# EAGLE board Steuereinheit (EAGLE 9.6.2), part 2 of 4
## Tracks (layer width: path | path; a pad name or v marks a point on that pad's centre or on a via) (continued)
GND  (via drill 0.35)  (1 unrouted) (continued)
  Top 0.152: SE_JK2.8 SE_JK2.7 17.7,55.35 17.7,54.63 16.81,53.75 v15.57,53.75 | v15.75,45.57 18.06,45.57 18.95,44.68 18.95,43.97 BR_NO3.8 | SE_JK7.8 18.95,101.22 17.88,101.22 SE_JK7.7 17.7,101.04 17.7,99.8 16.64,98.73 v15.57,98.73 | v17.53,97.49 18.06,97.49 18.95,96.6 18.95,95.88 SE_JK6.9 | v16.28,108.86 18.06,108.86 18.95,107.97 18.95,107.26 SE_JK7.9 | SE_JK12.7 17.88,66.9 18.95,66.9 SE_JK12.8 19.13,66.9 21.62,66.9 23.75,69.04 23.75,70.64 21.62,72.77 19.13,72.77 SE_JK12.9 18.95,72.95 18.95,73.66 18.06,74.55 v15.57,74.55 | v15.57,79.88 18.95,83.26 18.95,84.33 SE_JK5.9 | PL_XR.11 42.6,24.77 43.66,24.77 PL_XR.10 43.84,24.77 43.84,25.3 44.2,25.65 | 44.2,25.65 46.33,27.79 46.33,29.92 M_OR1.7 | PL_XR.7 46.33,18.36 46.33,17.83 45.62,17.12 43.31,17.12 42.6,17.83 42.6,18.36 PL_XR.4 42.6,18.54 42.6,19.25 v43.48,20.14 | v43.48,26.37 44.2,25.65 | v44.2,56.95 45.97,56.95 46.86,56.06 46.86,55.35 BR_AA4.7 | 52.38,108.69 52.55,108.86 SE_BF1.3 52.38,108.69 | 52.38,108.69 50.95,107.26 50.95,105.13 52.2,103.89 52.55,103.89 SE_BF2.3 | 52.55,112.6 52.55,112.06 51.66,111.18 51.66,109.4 52.38,108.69 | 52.55,112.6 52.55,113.84 SE_BF0.3 | SE_AN2.7 48.28,101.22 48.82,101.75 50.06,101.75 50.42,101.4 50.42,100.15 51.66,98.91 52.55,98.91 SE_BF3.3 52.55,98.73 v52.55,97.84 | v52.73,77.39 52.73,78.28 SE_BF7.3 | v52.73,112.6 52.55,112.6 | SE_JK10.12 30.51,95.88 30.51,96.42 31.22,97.13 33.53,97.13 34.24,96.42 34.24,95.88 SE_JK10.9 34.24,95.71 34.24,91.97 | SE_JK9.12 30.51,84.33 30.51,83.62 31.22,82.91 33.53,82.91 34.24,83.62 34.24,84.33 SE_JK9.9 34.24,84.51 34.24,85.22 31.75,87.71
  Top 0.152: SE_JK6.7 17.88,89.66 18.95,89.66 SE_JK6.8 19.13,89.48 21.08,89.48 23.39,87.17 28.91,87.17 29.26,87.53 | 29.26,87.53 29.26,89.48 SE_JK10.4 | 29.26,87.53 29.62,87.17 v30.86,87.17 31.22,87.17 31.75,87.71 | 31.75,87.71 32.99,88.95 32.99,89.48 SE_JK10.7 33.17,89.66 34.24,89.66 | 34.24,89.66 34.24,91.97 | 34.24,89.66 SE_JK10.8 | BR_NO4.8 48.28,66.9 48.28,70.99 49.35,72.06 49.35,77.04 48.28,78.1 SE_JK8.8 48.11,78.28 47.04,78.28 SE_JK8.7 46.86,78.28 46.86,78.99 46.15,79.7 44.55,79.7 | 52.55,88.42 52.2,88.06 | 52.2,88.06 50.77,86.64 50.77,84.86 52.02,83.62 52.55,83.62 SE_BF6.3 | 51.31,91.44 52.55,92.69 52.55,93.57 SE_BF4.3 | 51.31,91.44 51.31,89.66 52.55,88.42 | 52.55,88.42 SE_BF5.3 | 48.28,85.75 48.28,89.48 SE_AN1.7 48.11,89.66 48.11,90.37 46.68,91.8 46.68,92.86 47.22,93.4 48.82,93.4 50.77,91.44 51.31,91.44 | 48.28,85.75 48.28,84.51 SE_JK8.9 | SE_JK9.7 33.17,78.28 34.24,78.28 SE_JK9.8 34.42,78.1 35.66,78.1 | 44.55,79.7 44.02,79.7 43.31,78.99 43.31,78.28 SE_JK8.4 43.13,78.1 43.13,77.57 42.06,76.5 38.68,76.5 37.08,78.1 35.66,78.1 | 44.55,79.7 44.55,84.33 SE_JK8.12 44.55,84.51 44.55,85.04 45.26,85.75 48.28,85.75 | 34.24,91.97 35.31,91.97 35.66,91.62 35.66,78.1 | 52.2,88.06 v52.73,87.53 | X2.M2 9.53,8.59 X2.M3 9.35,8.76 9.35,10.01 7.04,12.32 C9.1 6.86,12.5 5.79,13.56 5.79,17.12 9.17,20.5 10.06,20.5 FT232.7 | 18.95,18.19 19.66,18.19 20.19,18.72 20.19,19.43 19.66,19.96 18.95,19.96 | 18.95,18.19 17.88,18.19 FT232.18 | 18.95,19.96 17.88,19.96 FT232.21 | 18.95,19.96 18.95,22.28 18.77,22.45 17.88,22.45 FT232.25 17.88,22.63 17.88,23.16 FT232.26 17.7,23.34 v15.39,23.34
  Top 0.152: X2.M1 18.41,8.59 X2.M4 | X2.5 15.57,8.76 18.41,8.76 X2.M4 | 18.95,13.74 18.95,9.12 18.59,8.76 X2.M4 | 18.95,13.74 18.95,18.19 | X2.M1 X2.M2 | X2.M2 | X2.M1 | 31.75,18.54 32.46,19.25 32.99,19.25 | 32.99,19.25 33.53,19.25 34.24,18.54 34.24,18.01 SE_N01.8 | SE_JK1.7 17.88,30.1 18.95,30.1 SE_JK1.8 19.13,29.92 21.08,29.92 25.53,25.48 26.06,25.48 26.77,24.77 | 26.77,24.77 26.77,24.05 SE_N01.15 26.77,24.77 | 26.77,24.77 27.48,25.48 29.62,25.48 30.33,24.77 | 30.33,24.77 30.33,24.05 SE_N01.12 30.33,24.77 | 31.04,25.48 32.28,25.48 32.99,24.77 32.99,24.05 SE_N01.10 32.99,23.88 32.99,19.25 | 30.33,24.77 31.04,25.48 | 30.86,27.61 26.77,27.61 22.86,31.52 22.86,34.54 21.44,35.97 19.13,35.97 SE_JK1.9 | 30.86,27.61 33.35,27.61 34.24,28.5 34.24,29.92 SE_AN3.7 | CLKNO.7 46.86,12.14 29.79,12.14 29.26,12.68 MCLKC.2 29.08,12.85 28.19,13.74 18.95,13.74 | v30.86,27.96 30.86,27.61 | v30.86,25.65 31.04,25.48 | 31.75,102.46 32.28,102.46 32.99,101.75 32.99,101.22 SE_JK11.7 33.17,101.22 34.24,101.22 SE_JK11.8 | 31.75,102.46 29.97,102.46 29.26,101.75 29.26,101.22 SE_JK11.4 | SE_JK11.9 34.24,107.09 34.24,106.55 33.53,105.84 31.22,105.84 30.51,106.55 30.51,107.09 SE_JK11.12 30.51,107.26 v30.51,108.86 | v31.75,102.82 31.75,102.46 | SE_JK5.7 17.88,78.28 18.95,78.28 SE_JK5.8 19.13,78.1 20.55,78.1 22.68,75.97 27.66,75.97 28.91,77.22 | 28.91,77.22 29.08,77.39 29.08,78.1 SE_JK9.4 28.91,77.22 | SE_JK3.7 SE_JK3.8 34.42,55.35 34.42,61.39 SE_JK3.9 34.24,61.57 34.24,62.1 32.64,63.7 v30.86,63.7 | SE_JK4.8 34.24,66.9 33.17,66.9 SE_JK4.7 32.99,66.9 v32.99,68.5 | v31.57,42.19 33.17,42.19 34.24,43.26 34.24,43.79 BR_OR1.7
  Top 0.152: v32.99,71.17 33.17,71.17 34.24,72.24 34.24,72.77 SE_JK4.9 | v29.62,76.5 28.91,77.22 | BR_JK4.7 144.3,45.21 145.36,45.21 BR_JK4.8 145.54,45.21 145.54,47.35 | 145.54,47.35 145.54,51.26 BR_JK4.9 | 141.45,42.01 140.39,43.08 140.39,45.03 BR_JK4.4 140.39,45.21 140.39,46.99 141.45,48.06 | 141.45,42.01 141.45,40.06 BR_JK8.12 141.45,39.88 141.45,37.57 139.14,35.26 | 141.45,48.06 141.45,51.26 BR_JK4.12 | 145.54,47.35 142.16,47.35 141.45,48.06 | BR_JK7.12 127.76,40.06 127.76,40.59 128.47,41.3 130.61,41.3 131.32,40.59 131.32,40.06 BR_JK7.9 131.32,39.88 131.32,37.74 129.72,36.14 | 127.23,35.26 128.12,36.14 129.72,36.14 | 127.23,35.26 126.52,34.54 126.52,33.83 BR_JK7.4 | 129.72,36.14 130.07,35.79 130.07,33.83 BR_JK7.7 130.25,33.83 131.32,33.83 BR_JK7.8 131.5,33.83 134.7,33.83 136.12,35.26 139.14,35.26 | BR_JK8.9 145.54,39.88 145.54,33.83 BR_JK8.8 145.36,33.83 144.3,33.83 BR_JK8.7 144.12,33.66 144.12,33.12 143.41,32.41 141.1,32.41 140.39,33.12 140.39,33.66 BR_JK8.4 140.21,33.83 140.21,34.54 139.5,35.26 139.14,35.26 | 144.83,82.02 144.83,82.55 145.54,83.26 145.54,88.77 144.83,89.48 PC_AN10.7 | 144.83,82.02 144.83,78.28 PC_AN11.7 | v142.88,99.44 143.76,99.44 144.65,100.33 144.65,101.04 PC_AN5.7 | 144.83,82.02 142.7,82.02 v141.99,82.73 | 138.43,67.44 137.72,68.15 136.65,68.15 135.41,66.9 130.96,66.9 PC_AN8.7 | 138.43,67.44 PC_NO1.2 138.43,66.9 | 140.92,67.44 140.92,66.9 PC_NO1.4 140.92,67.44 | 140.92,67.44 140.21,68.15 139.14,68.15 138.43,67.44 | v142.52,56.95 142.52,57.12 143.23,57.84 144.12,57.84 145.9,56.06 145.9,55.35 PC_NO2.8 | v142.52,63.35 143.23,63.35 145.9,66.02 145.9,66.73 PC_NO1.8
  Top 0.152: 140.92,67.44 141.99,68.5 v142.52,68.5 | v141.99,42.01 141.45,42.01 | v145.36,22.45 144.83,22.99 144.83,23.7 RE_BF3.3 | v132.21,22.63 132.21,23.7 WR_BF3.3 | 145.36,13.74 144.83,13.74 RE_BF1.3 145.36,13.74 | 145.36,13.74 145.9,14.28 145.9,17.65 144.83,18.72 RE_BF2.3 | 132.21,3.25 132.21,8.41 WR_BF0.3 | 132.21,3.25 133.99,1.47 139.68,1.47 141.1,2.9 141.1,5.03 144.65,8.59 RE_BF0.3 144.83,8.59 145.19,8.59 145.9,9.3 145.9,10.72 145.36,11.25 145.36,12.32 | 125.81,2.54 125.81,6.45 132.03,12.68 132.03,13.56 WR_BF1.3 | 125.81,2.54 126.52,1.83 130.78,1.83 132.21,3.25 | 132.03,16.94 132.03,18.72 WR_BF2.3 | 132.03,16.94 123.32,8.23 123.32,2.54 | 123.32,2.54 124.03,1.83 125.09,1.83 125.81,2.54 | 123.32,2.54 122.61,1.83 119.05,1.83 118.16,2.72 118.16,7.52 126.87,16.23 126.87,18.36 BR_AN2.7 | 145.36,12.32 145.36,13.74 | 132.03,16.94 v132.21,16.94 | 145.36,12.32 v145.54,12.32 | 129.18,102.82 129.72,102.82 130.78,101.75 130.78,101.22 PC_AN9.7 | 129.18,102.82 122.96,102.82 121.36,101.22 115.67,101.22 PC_JK5.8 115.49,101.22 115.49,101.75 114.43,102.82 v113,102.82 | v128.12,91.26 129.9,91.26 130.78,90.37 130.78,89.66 PC_AN6.7 | v129.18,103.18 129.18,102.82 | BR_JK3.4 126.34,45.21 126.34,48.95 127.58,50.19 127.58,51.26 BR_JK3.12 127.76,51.44 127.76,52.15 128.3,52.68 | BR_JK3.7 130.25,45.21 131.32,45.21 BR_JK3.8 131.5,45.21 131.5,51.26 BR_JK3.9 131.32,51.44 130.96,51.79 130.96,52.68 | 130.96,52.68 130.96,55.35 PC_AN1.7 | 130.96,52.68 128.3,52.68 | v127.94,76.33 129.54,76.33 130.78,77.57 130.78,78.1 PC_AN7.7 | v127.94,53.04 128.3,52.68 | 127.23,35.26 127.05,35.26 v126.87,35.43 | 98.25,51.08 98.6,51.44 100.91,51.44
  Top 0.152: 98.25,51.08 97.89,50.72 97.89,50.19 BR_JK2.12 | 100.91,51.44 101.45,50.9 101.45,50.19 BR_JK2.9 101.45,50.01 101.45,46.99 99.67,45.21 | 100.91,51.44 101.45,51.97 101.45,55.35 BR_NO1.8 | BR_JK1.12 85.09,48.59 85.98,47.7 87.76,47.7 88.82,48.77 | 88.82,48.77 88.82,50.01 BR_JK1.9 | 99.67,45.21 100.2,44.68 100.2,43.97 BR_JK2.7 100.38,43.97 101.45,43.97 BR_JK2.8 | 99.67,45.21 99.49,45.39 97.36,45.39 96.65,44.68 96.65,43.97 BR_JK2.4 96.47,43.79 96.47,43.26 95.4,42.19 92.02,42.19 91.67,42.55 91.67,45.92 88.82,48.77 | v99.85,91.26 100.56,91.26 101.45,90.37 101.45,89.66 PC_JK2.8 | v99.31,103 100.38,103 101.45,101.93 101.45,101.22 PC_JK1.8 | BR_NO1.2 93.98,56.06 96.11,58.19 | 96.11,58.19 97,59.08 101.09,59.08 102.34,60.33 102.34,64.77 PC_AN3.7 | 97.89,37.03 97.89,38.63 BR_JK6.12 | 97.89,37.03 98.6,36.32 99.85,36.32 101.45,37.92 101.45,38.63 BR_JK6.9 | v97,20.14 97.71,20.85 99.49,20.85 100.2,20.14 100.2,18.54 BR_AN4.7 | v97.54,37.03 97.89,37.03 | 96.11,58.19 97.36,56.95 v97.54,56.95 | 98.25,51.08 97.71,51.61 v97.71,51.79 | BR_OR7.11 111.23,38.63 111.23,39.34 v112.12,40.23 113.72,41.83 115.85,41.83 116.74,42.72 116.74,52.15 115.67,53.21 115.67,55.35 PC_AN4.7 | 112.47,22.99 112.47,21.57 114.78,19.25 114.78,18.54 BR_AN7.7 | 112.47,22.99 112.47,24.59 BR_AN7.10 | BR_OR6.7 115.49,43.79 115.49,43.26 114.78,42.55 112.47,42.55 111.76,43.26 BR_OR6.4 111.76,45.21 v112.12,45.57 | v112.12,22.99 112.47,22.99 | v114.96,91.26 115.49,90.73 115.49,89.66 PC_JK6.8 | PC_JK3.8 101.62,78.1 103.94,78.1 106.07,75.97 118.16,75.97 118.87,76.68 118.87,77.39 118.16,78.1 115.67,78.1 PC_JK7.8 115.49,78.28 115.49,78.99 114.61,79.88 v112.12,79.88
  Top 0.152: v112.12,68.5 114.43,68.5 115.49,67.44 115.49,66.9 PC_JK4.8 | BR_JK5.12 85.09,37.92 85.62,37.39 | 85.62,37.39 85.8,37.21 88.11,37.21 88.82,37.92 88.82,38.63 BR_JK5.9 89,38.63 89,43.79 | 96.65,33.3 96.65,32.59 BR_JK6.4 | 96.65,33.3 97.18,33.83 99.67,33.83 100.2,33.3 100.2,32.59 BR_JK6.7 100.38,32.59 101.45,32.59 BR_JK6.8 101.62,32.41 103.05,30.99 111.58,30.99 112.65,29.92 114.96,29.92 115.32,30.28 115.32,30.99 114.96,31.34 114.96,32.41 BR_OR7.7 114.78,32.59 114.78,33.3 113.89,34.19 v112.12,34.19 | 89,43.79 90.25,43.79 90.78,43.26 90.78,39.52 92.02,38.28 92.02,36.86 93.45,35.43 94.51,35.43 96.65,33.3 | 89,43.79 BR_JK1.8 | 96.65,33.3 BR_JK6.4 | 84.73,20.85 85.98,20.85 87.58,19.25 87.58,18.54 BR_AN3.7 | 84.73,20.85 80.29,20.85 77.98,18.54 74.95,18.54 BR_OR4.7 | v84.73,20.14 84.73,20.85 | 85.62,37.39 85.62,37.21 v85.45,37.03 | v58.06,68.5 58.78,69.22 59.66,69.22 60.91,67.97 60.91,66.9 BR_OR2.7 | v56.29,16.76 58.6,16.76 59.66,17.83 59.66,18.36 M_NO1.8 | BR_JK5.8 88.82,32.59 87.76,32.59 BR_JK5.7 87.58,32.59 87.58,33.12 86.87,33.83 84.56,33.83 83.84,33.12 83.84,32.59 BR_JK5.4 83.67,32.41 83.67,30.63 | 77.44,31.7 80.11,29.03 83.31,29.03 83.67,29.39 83.67,30.63 | 77.44,31.7 76.73,32.41 76.2,32.41 BR_NO2.8 | 47.04,45.57 47.04,43.97 BR_AA1.7 | 47.04,45.57 47.57,46.1 49.53,46.1 49.89,45.75 59.13,45.75 59.66,46.28 60.38,46.28 60.91,45.75 | 60.91,45.75 60.91,43.97 BR_AA2.7 61.09,43.79 61.09,41.83 62.86,40.06 PLC.2 62.86,34.54 67.31,30.1 v72.11,30.1 75.84,30.1 77.44,31.7 | 60.91,45.75 62.51,47.35 62.51,47.52 62.69,47.7 62.69,51.08 61.09,52.68 61.09,55.35 BR_AA3.7
  Top 0.152: 66.06,111.71 66.06,110.82 SP_BF1.3 | 66.06,111.71 68.02,113.66 68.02,114.38 66.6,115.8 66.06,115.8 SP_BF0.3 | v65.53,81.66 65.89,81.31 65.89,80.42 SP_BF7.3 | v64.82,86.64 65.89,85.57 SP_BF6.3 | 66.06,111.71 65.53,111.71 v65.18,112.06 | 67.67,97.31 66.06,95.71 SP_BF4.3 | 67.67,99.44 67.67,97.31 | 67.67,99.44 66.6,100.51 66.06,100.51 SP_BF3.3 | 67.67,99.44 69.09,100.86 69.09,103 66.42,105.66 66.06,105.66 SP_BF2.3 65.89,105.84 64.82,106.91 v63.58,106.91 | 87.58,87.88 69.98,87.88 67.49,90.37 66.06,90.37 SP_BF5.3 | 87.58,87.88 88.11,88.42 88.11,89.84 86.51,91.44 M48Z08.20 84.56,91.44 81,95 70.51,95 68.2,97.31 67.67,97.31 | 86.87,65.3 87.58,66.02 87.58,66.73 PC_AN2.7 | 86.87,65.3 86.51,64.95 81.36,64.95 81,64.59 78.87,64.59 76.73,66.73 74.95,66.73 BR_AN6.7 | 74.95,45.57 74.95,46.99 78.16,50.19 78.16,51.08 79.76,52.68 82.25,52.68 82.42,52.86 87.05,52.86 87.58,53.39 87.58,55.17 BR_OR5.7 87.76,55.35 88.82,56.41 88.82,63.35 86.87,65.3 | 74.95,45.57 74.95,43.97 BR_AN1.7 | v72.11,53.39 72.47,53.04 74.07,53.04 74.78,53.75 74.78,55.35 BR_AN5.7 | v72.82,45.57 74.95,45.57 | 87.58,87.88 88.47,87 88.47,83.8 87.05,82.37 74.78,82.37 71.22,78.82 M48Z08.14 | 83.67,30.63 v84.73,30.63 | v97,30.81 97,32.05 96.65,32.41 BR_JK6.4 | 47.04,45.57 v44.37,45.57
  Bottom 0.152: C10.1 13.97,20.68 15.39,22.1 v15.39,23.34 15.39,32.94 C14.2 15.57,33.12 15.57,45.75 | 15.57,46.99 v15.57,53.75 15.57,58.37 C15.2 15.57,58.55 15.57,69.75 C32.2 15.57,69.93 v15.57,74.55 v15.57,79.88 15.57,81.13 C81.2 15.57,81.31 15.57,92.69 C18.2 15.57,92.86 15.57,97.49 | 15.57,46.99 15.57,45.75 | 15.57,46.99 C35.2 | 15.57,45.75 v15.75,45.57 | 15.57,97.49 v15.57,98.73 15.57,104.06 C17.2 15.57,104.24 15.57,108.15 v16.28,108.86 | 15.57,97.49 v17.53,97.49 | C82.2 45.44,104.06 45.44,92.86 C83.2 45.26,92.69 45.09,92.51 45.09,81.48 44.91,81.31 C57.2 44.73,81.13 44.73,69.93 C43.2 44.73,69.75 44.73,59.08 44.2,58.55 C68.2 44.2,58.37 v44.2,56.95 44.2,46.99 C67.2 44.02,46.99 44.02,45.57 | 44.02,45.57 44.02,33.48 43.66,33.12 C72.2 43.48,32.94 v43.48,26.37 43.48,21.74 C3.2 43.48,21.57 v43.48,20.14 46.86,16.76 46.86,12.14 CLKNO.7 47.04,11.96 47.04,10.36 | C59.2 53.98,78.28 53.62,78.28 v52.73,77.39 52.73,82.19 | 52.73,82.19 53.98,83.44 C60.2 | 52.73,87.17 53.98,88.42 C61.2 | 52.73,82.19 52.73,87.17 | 52.73,92.33 53.98,93.57 C88.2 | 52.73,87.17 v52.73,87.53 52.73,92.33 | 52.73,97.49 C62.2 | 52.73,92.33 52.73,97.49 | 52.73,102.46 53.98,103.71 C63.2 | 52.73,97.49 52.73,97.84 | 52.73,97.84 52.73,102.46 | 52.73,107.62 52.55,107.44 52.55,102.64 52.73,102.46 | 52.73,107.62 53.98,108.86 C89.2 | 52.73,107.62 v52.73,112.6 53.98,113.84 C86.2 | 52.73,97.84 v52.55,97.84 | 47.04,10.36 52.2,10.36 54.15,8.41 C12.2 | 47.04,10.36 47.04,4.5 CLKNO.8 | MCLKC.2 29.26,12.85 29.26,19.43 30.68,20.85 C13.2 30.86,21.03 v30.86,25.65 v30.86,27.96 30.86,32.41 31.39,32.94 C16.2 31.57,33.12 v31.57,42.19 31.57,46.99 C94.2 31.39,46.99 31.22,47.17 31.22,58.01 30.86,58.37 C84.2 30.86,58.55 v30.86,63.7 30.86,69.75 C33.2 30.86,69.93 30.86,71.35
  Bottom 0.152: 30.86,102.82 30.86,104.06 C55.2 30.68,104.24 30.68,108.69 v30.51,108.86 | 30.86,102.82 30.86,92.86 C56.2 30.86,92.69 v30.86,87.17 30.86,81.31 C31.2 30.86,81.13 30.86,76.5 | 30.86,102.82 v31.75,102.82 | 30.86,71.35 30.86,76.5 | 30.86,71.35 32.46,71.35 32.64,71.17 v32.99,71.17 v32.99,68.5 | 30.86,76.5 v29.62,76.5 | 141.99,99.44 141.99,92.86 C24.2 141.99,92.69 v141.99,82.73 141.99,81.31 C25.2 141.81,81.13 141.45,80.77 141.45,70.99 142.52,69.93 C26.2 142.52,69.75 v142.52,68.5 v142.52,63.35 142.52,58.55 C27.2 142.52,58.37 v142.52,56.95 142.52,48.95 141.99,48.41 C53.2 141.99,48.23 v141.99,42.01 141.99,36.86 C52.2 | 141.99,99.44 141.99,104.06 C28.2 | 141.99,99.44 v142.88,99.44 | v145.36,22.45 145.9,22.99 145.9,23.7 C42.2 146.08,23.7 147.14,22.63 147.14,17.65 | 147.14,12.5 147.14,9.65 146.08,8.59 C91.2 | 147.14,12.5 146.08,13.56 C92.2 145.9,13.56 145.54,13.21 v145.54,12.32 | 147.14,17.65 146.08,18.72 C66.2 | 147.14,12.5 147.14,17.65 | 132.21,12.5 132.21,9.65 133.27,8.59 C64.2 | 132.21,12.5 133.27,13.56 C90.2 | v132.21,22.63 133.27,23.7 C65.2 | 132.21,19.61 132.56,19.61 133.27,18.9 C41.2 | v132.21,22.63 132.21,19.61 | 132.21,19.61 v132.21,16.94 132.21,12.5 | v129.18,103.18 128.12,104.24 C29.2 127.94,104.06 127.94,92.86 C23.2 128.12,92.69 v128.12,91.26 127.94,91.08 127.94,81.31 C22.2 127.94,81.13 v127.94,76.33 127.94,69.93 C21.2 127.94,69.75 127.94,58.55 C54.2 127.94,58.37 v127.94,53.04 127.94,48.41 C8.2 127.94,48.23 127.94,36.86 C77.2 | 126.87,35.26 127.94,36.32 127.94,36.68 C77.2 | 126.87,35.26 124.38,32.77 124.38,21.92 124.21,21.74 C78.2 | v132.21,22.63 128.12,26.72 128.12,36.68 C77.2
  Bottom 0.152: 126.87,35.26 v126.87,35.43 | 98.07,91.26 98.07,92.69 C19.2 98.07,92.86 98.07,104.06 C79.2 98.25,104.06 v99.31,103 | 98.07,91.26 98.07,81.31 C49.2 98.07,81.13 97.71,80.77 97.71,69.57 | 98.07,91.26 v99.85,91.26 | 97.71,58.9 98.07,58.55 C48.2 97.71,58.9 | 97.71,69.57 97.71,58.9 | 97.71,69.57 97.54,69.75 C50.2 97.71,69.57 | 97.18,30.81 97.18,34.54 97.54,34.9 | 97.18,30.81 97.18,21.92 97,21.74 C6.2 97,21.57 v97,20.14 | 97.54,34.9 98.07,35.43 C74.2 97.54,34.9 | 97.54,34.9 v97.54,37.03 97.54,46.99 | 97.71,58.9 97.54,58.73 v97.54,56.95 97.54,51.79 | 97.54,46.99 97.54,51.79 | 97.54,46.99 C75.2 | 97.54,51.79 v97.71,51.79 | C34.2 112.12,21.74 v112.12,22.99 v112.12,34.19 112.12,35.43 C80.2 112.12,35.61 v112.12,40.23 v112.12,45.57 112.12,46.99 | 112.12,102.82 112.12,104.06 C30.2 | 112.12,102.82 112.12,92.86 C20.2 112.12,92.69 112.12,91.62 | v114.96,91.26 114.61,91.62 112.12,91.62 | 112.12,59.08 112.65,58.55 C7.2 112.12,59.08 | 112.12,59.08 v112.12,68.5 112.12,69.75 C76.2 112.12,69.93 v112.12,79.88 112.12,81.13 C51.2 112.12,81.31 112.12,91.62 | 112.12,59.08 112.12,46.99 | 112.12,46.99 C95.2 | C71.2 84.73,69.75 84.73,58.55 C2.2 84.91,58.37 85.27,58.01 85.27,46.99 C45.2 85.45,46.99 v85.45,37.03 85.45,35.61 C47.2 85.27,35.43 84.73,34.9 v84.73,30.63 84.73,21.74 C5.2 84.73,21.57 v84.73,20.14 84.73,13.03 82.6,10.9 MCLKR4.1 | C69.2 58.06,69.75 v58.06,68.5 58.06,58.55 C11.2 58.06,58.37 58.06,46.99 | 57.35,35.43 57.35,46.28 58.06,46.99 | 57.35,35.43 57.35,22.81 56.29,21.74 C4.2 56.29,21.57 v56.29,16.76 | 58.06,46.99 C93.2 | 57.35,35.43 62.86,35.43 PLC.2 | 64.82,80.95 v65.53,81.66 | 64.82,80.95 64.82,80.42 C36.2 64.82,80.95
  Bottom 0.152: C40.2 64.82,85.57 v64.82,86.64 63.58,87.88 | 63.58,89.31 64.64,90.37 C39.2 | 63.58,87.88 63.58,89.31 | 63.58,94.46 64.64,95.53 C38.2 | 63.58,89.31 63.58,94.46 | 63.58,99.44 64.64,100.51 C37.2 | 63.58,94.46 63.58,99.44 | 63.58,104.6 64.64,105.66 C58.2 | 63.58,99.44 63.58,104.6 | 63.58,109.93 63.93,109.93 64.64,110.64 C87.2 64.82,110.82 64.82,111.71 v65.18,112.06 | 63.58,104.6 v63.58,106.91 63.58,109.93 | 63.58,109.93 63.58,114.73 64.64,115.8 C85.2 | 64.82,80.95 63.58,82.19 63.58,87.88 | GND.1 73.53,4.32 73.53,18.36 72.11,19.79 72.11,21.57 C73.2 72.11,21.74 v72.11,30.1 72.11,33.3 72.64,33.83 72.64,35.43 C46.2 72.64,35.61 72.64,40.06 72.82,40.23 v72.82,45.57 72.82,46.28 72.11,46.99 | M48Z08.14 71.22,78.64 71.22,70.64 71.93,69.93 C44.2 72.11,69.75 72.11,58.55 C70.2 72.11,58.37 v72.11,53.39 72.11,46.99 | 72.11,46.99 C1.2 | v97,30.81 97.18,30.81 | 112.12,102.82 v113,102.82 | v44.37,45.57 44.02,45.57
GND2
  Top 0.152: BR_JK1.4 83.84,43.79 83.84,41.48 84.2,41.12 85.98,41.12 87.58,42.72 87.58,43.79 BR_JK1.7
M_CARRYFLAG  (via drill 0.35)
  Top 0.152: v67.67,41.12 68.56,42.01 68.56,43.79 BR_AN1.2 | v91.31,13.03 92.02,13.03 99.31,5.74 101.98,5.74 105.36,2.36 113.36,2.36 114.78,3.79 CARRY.1
  Route15 0.152: v67.67,41.12 68.2,41.12 74.07,35.26 76.73,35.26 82.25,29.74 82.25,29.39 83.13,28.5 83.49,28.5 87.58,24.41 87.58,16.76 v91.31,13.03
M_CLK  (via drill 0.35)
  Top 0.152: 92.56,47.7 92.2,48.06 92.2,48.59 89.36,51.44 84.56,51.44 83.84,50.72 83.84,50.19 BR_JK1.13 | 92.56,47.7 94.87,47.7 96.47,49.3 96.47,50.01 BR_JK2.13 96.65,50.19 96.65,51.79 97.36,52.5 v98.96,52.5 | 92.56,47.7 92.02,47.17 92.02,42.72 92.2,42.55 94.51,42.55 95.22,43.26 95.22,43.79 BR_JK2.3 95.22,43.97 95.22,45.21 v94.87,45.57 | v117.8,54.28 117.8,56.06 114.43,59.44 114.43,61.39 PC_AN4.9 | CLK.1 77.44,3.96 76.38,5.03 72.64,5.03 69.98,2.36 52.02,2.36 50.95,3.43 50.95,14.45 M_CLK.1 50.95,14.63 50.06,15.52 49.71,15.52 | 49.71,15.52 33.71,15.52 | 33.71,15.52 25.35,15.52 21.62,19.25 21.62,22.28 18.59,25.3 16.64,25.3 12.72,29.21 12.72,29.92 SE_JK1.3 | v33.71,33.12 30.51,33.12 29.26,34.37 29.26,35.97 SE_AN3.12 | 33.71,15.52 v33.71,16.23 | v49.71,25.48 50.24,26.01 52.55,26.01 53.26,25.3 53.26,24.77 M_NO1.14 | 49.71,15.52 v49.71,19.07
  Route2 0.152: v94.87,45.57 86.16,36.86 86.16,36.68 81,31.52 79.22,31.52 v77.09,29.39
  Route15 0.152: v117.8,54.28 116.38,54.28 114.61,52.5 111.94,52.5 110.52,51.08 100.38,51.08 v98.96,52.5
  Bottom 0.152: v33.71,16.23 v33.71,33.12 | v49.71,19.07 v49.71,25.48 | v77.09,29.39 77.44,29.03 77.44,3.96 CLK.1
M_PC_SET  (via drill 0.35)
  Top 0.152: PC_AN9.2 124.56,101.22 124.56,101.75 125.27,102.46 128.83,102.46 129.54,101.75 PC_AN9.6 129.54,100.51 130.43,99.62 131.32,99.62 131.5,99.8 131.5,103.89 | PC_AN9.13 124.56,107.26 124.56,107.97 125.27,108.69 128.65,108.69 129.54,107.8 PC_AN9.9 129.54,106.55 131.5,104.6 131.5,103.89 | PC_AN8.6 PC_AN8.9 129.54,74.37 v129.72,74.55 | v129.54,79.88 PC_AN7.6 | v129.54,82.02 PC_AN7.9 PC_AN6.6 | PC_AN10.13 138.43,96.42 137.01,97.84 130.96,97.84 v130.43,98.37 | v130.43,103.89 131.5,103.89 | 124.56,96.6 124.56,95.88 PC_AN6.13 124.56,96.6 | 124.56,96.6 125.09,97.13 128.83,97.13 | 128.83,97.13 129.54,96.42 PC_AN6.9 129.54,95.17 132.39,92.33 136.47,92.33 138.43,90.37 | 122.43,92.33 116.74,92.33 116.38,91.97 116.38,90.19 117.8,88.77 118.87,88.77 121.18,86.46 123.14,86.46 124.38,85.22 124.38,84.51 PC_AN7.13 124.38,84.33 v124.38,82.73 | 122.43,92.33 124.38,90.37 124.38,89.66 PC_AN6.2 | 124.56,96.6 124.21,96.6 123.67,97.13 122.61,97.13 122.43,96.95 122.43,92.33 | PC_AN5.13 138.43,107.8 139.32,108.69 142.7,108.69 143.41,107.97 143.41,107.26 PC_AN5.9 143.59,107.09 v143.59,102.82 143.59,101.22 PC_AN5.6 | PC_AN11.2 138.43,78.82 140.21,80.59 142.52,80.59 143.41,79.7 143.41,78.28 PC_AN11.6 143.59,78.1 143.59,77.57 144.3,76.86 145.36,76.86 146.25,77.75 146.25,90.02 144.48,91.8 v143.41,91.8 142.7,91.08 | 138.43,90.37 PC_AN10.2 138.43,89.66 | 138.43,90.37 140.03,91.97 141.81,91.97 142.7,91.08 | 142.7,91.08 143.41,90.37 143.41,89.66 PC_AN10.6 143.59,89.48 143.59,84.51 PC_AN11.9 | v143.41,94.11 143.41,95.71 PC_AN10.9 | 128.83,97.13 v129.18,97.49 | v62.86,17.65 61.27,16.05 55.75,16.05 54.69,17.12 54.69,18.36 M_NO1.4
  Top 0.152: v122.25,72.24 122.25,73.84 122.78,74.37 123.67,74.37 124.38,73.66 124.38,72.95 PC_AN8.13 | v123.5,68.5 124.38,67.62 124.38,66.9 PC_AN8.2 | v122.96,79.88 123.5,79.88 124.38,78.99 124.38,78.28 PC_AN7.2
  Route2 0.152: v62.86,17.65 68.91,17.65 76.2,24.94 79.4,24.94 82.96,28.5 84.38,28.5 91.67,35.79 91.67,37.57 92.2,38.1 92.2,41.12 118.16,67.08 118.69,67.08 120.83,69.22 120.83,70.81 v122.25,72.24
  Bottom 0.152: 129.54,97.49 v130.43,98.37 v130.43,103.89 | 129.54,97.49 v129.54,82.02 v129.54,79.88 129.54,74.73 v129.72,74.55 | v143.41,91.8 v143.41,94.11 143.59,94.28 v143.59,102.82 | v129.18,97.49 129.54,97.49 | v123.5,68.5 123.14,68.86 123.14,71.35 | v122.25,72.24 123.14,71.35 | 123.14,71.35 123.14,79.7 v122.96,79.88 122.96,81.31 v124.38,82.73
M_RE_N0  (via drill 0.35)
  Top 0.152: v147.5,24.77 147.32,24.59 147.32,23.88 RE_BF3.4 | v147.5,26.72 146.08,26.72 145.01,27.79 141.99,27.79 141.63,27.43 130.61,27.43 130.25,27.08 127.05,27.08 126.34,26.37 | 126.34,26.37 125.81,25.83 125.81,24.77 BR_AN2.9 | v73.71,65.13 73.71,66.73 BR_AN6.6 | 126.34,26.37 v126.16,26.37
  Route2 0.152: v104.47,37.03 104.65,37.21 105.72,37.21 116.56,26.37 v126.16,26.37
  Route15 0.152: v73.71,65.13 73.71,67.08 76.91,70.28 84.73,70.28 94.51,60.5 102.51,60.5 v104.47,58.55
  Bottom 0.152: v147.5,26.72 v147.5,24.77 | v104.47,37.03 v104.47,58.55
M_RE_N1  (via drill 0.35)
  Top 0.152: v146.25,21.92 146.25,20.32 147.14,19.43 147.14,18.9 RE_BF2.4 | v138.61,28.14 123.5,28.14 122.78,27.43 | 122.78,27.43 120.65,25.3 BR_AN2.13 | v79.22,69.57 78.33,70.46 75.49,70.46 73.71,72.24 73.71,72.77 BR_AN6.9 | v118.69,36.14 118.69,31.52 122.78,27.43
  Route2 0.152: v146.25,21.92 145.9,21.92 145.72,21.74 145.01,21.74 v138.61,28.14 | v79.22,69.57 85.45,69.57 87.22,67.79 v118.34,67.79
  Bottom 0.152: v118.34,67.79 118.69,67.44 v118.69,36.14
M_RE_N2  (via drill 0.35)
  Top 0.152: v148.21,14.63 147.32,13.74 RE_BF1.4 | v121.01,20.14 121.01,18.9 120.65,18.54 BR_AN2.2 | v65.71,70.99 66.24,71.53 66.24,73.84 66.78,74.37 67.84,74.37 68.56,73.66 68.56,72.95 BR_AN6.13
  Route2 0.152: v148.21,14.63 140.56,14.63 135.76,19.43 121.72,19.43 v121.01,20.14
  Route15 0.152: v62.86,41.12 62.86,40.06 71.04,31.88 77.8,31.88 81.53,28.14 83.31,28.14 86.51,24.94 86.51,13.39 87.58,12.32 111.94,12.32 119.76,20.14 v121.01,20.14
  Bottom 0.152: v65.71,70.99 63.22,68.5 63.22,43.79 62.86,43.43 v62.86,41.12
M_RE_N3  (via drill 0.35)
  Top 0.152: v119.41,31.88 121.01,30.28 145.01,30.28 150.52,24.77 150.52,11.43 147.68,8.59 147.32,8.59 RE_BF0.4 | v86.69,53.57 85.45,53.57 85.09,53.92 82.25,53.92 81.36,53.04 76.91,53.04 75.67,51.79 70.16,51.79 69.8,51.44 69.27,51.44 68.73,50.9 68.73,50.19 BR_AN1.13 68.56,50.01 68.56,49.48 67.67,48.59 66.95,48.59 64.64,50.9 64.64,60.68 68.56,64.59 68.56,66.73 BR_AN6.2
  Route15 0.152: v119.41,31.88 116.38,31.88 102.16,46.1 101.27,46.1 98.96,48.41 98.96,48.77 96.65,51.08 95.05,51.08 92.56,53.57 v86.69,53.57
M_SAMEFLAG  (via drill 0.35)
  Top 0.152: v87.94,41.3 87.4,40.77 84.02,40.77 82.96,41.83 74.95,41.83 73.71,43.08 73.71,43.79 BR_AN1.6 | v87.22,13.74 91.85,13.74 98.78,6.81 101.45,6.81 105.54,2.72 109.27,2.72 110.34,3.79 SMF.1
  Bottom 0.152: v87.94,41.3 87.22,40.59 v87.22,13.74
M_SETPCN0  (via drill 0.35)
  Top 0.152: v48.28,58.73 48.28,64.41 47.04,65.66 47.04,66.73 BR_NO4.7 | v142.16,79.88 142.16,78.28 PC_AN11.5 | v127.05,56.95 127.05,55.35 PC_AN1.4
  Route2 0.152: v48.28,58.73 49.53,58.73 58.24,67.44 60.38,67.44 65,72.06 68.56,72.06 73.89,77.39 91.14,77.39 102.51,88.77 122.25,88.77 125.45,91.97 129.01,91.97 138.43,82.55 138.43,82.37 140.21,80.59 141.45,80.59 v142.16,79.88
  Route15 0.152: v127.05,56.95 127.05,61.39 142.16,76.5 v142.16,79.88
M_SETPCN1  (via drill 0.35)
  Top 0.152: v44.02,65.13 44.37,65.48 44.37,66.73 BR_NO4.5 | v139.14,97.49 139.14,96.42 139.68,95.88 PC_AN10.12 | v124.21,53.75 124.74,53.75 125.63,54.63 125.63,55.35 PC_AN1.3
  Route2 0.152: v44.02,65.13 43.31,64.41 42.6,64.41 42.06,64.95 42.06,71.35 52.55,81.84 52.91,81.84 60.55,89.48 60.55,104.95 63.58,107.97 68.38,107.97 70.69,110.29 90.78,110.29 94.87,106.2 v118.34,106.2 131.14,106.2 133.99,103.35 135.41,103.35 139.14,99.62 v139.14,97.49
  Bottom 0.152: v124.21,53.75 120.29,57.66 120.29,104.24 v118.34,106.2
M_SETPCN2  (via drill 0.35)
  Top 0.152: v42.95,65.13 42.06,66.02 42.06,66.73 BR_NO4.3 | v140.39,91.26 141.28,91.26 142.16,90.37 142.16,89.66 PC_AN10.5 | v128.65,59.79 128.3,60.15 128.3,61.39 PC_AN1.10
  Route2 0.152: v42.95,65.13 42.95,66.19 55.75,78.99 55.75,80.59 59.66,84.51 59.66,87.88 60.91,89.13 60.91,96.24 61.62,96.95 61.62,105.49 61.98,105.84 70.51,105.84 71.22,105.13 83.84,105.13 86.33,102.64 96.29,102.64 101.62,97.31 107.67,97.31 113.36,91.62 114.07,91.62 114.78,92.33 139.32,92.33 v140.39,91.26
  Route15 0.152: v128.65,59.79 128.65,62.46 145.01,78.82 145.01,86.64 v140.39,91.26
M_SETPCN3  (via drill 0.35)
  Top 0.152: v133.27,62.1 132.39,62.99 127.94,62.99 127.05,62.1 127.05,61.57 PC_AN1.11 | v135.05,60.33 135.76,60.33 137.01,59.08 137.9,59.08 139.68,60.86 139.68,61.39 PC_NO2.14 | v125.27,105.49 125.63,105.84 125.63,107.09 PC_AN9.12
  Route2 0.152: v135.05,60.33 v133.27,62.1
  Bottom 0.152: v125.27,105.49 125.98,106.2 131.85,106.2 131.85,78.46 133.27,77.04 v133.27,62.1
M_SETPCN4  (via drill 0.35)
  Top 0.152: v78.51,71.53 79.58,70.46 80.64,70.46 82.42,68.68 82.42,66.9 PC_AN2.3 | 133.1,114.73 139.14,114.73 150.52,103.35 150.52,62.99 146.43,58.9 145.54,58.9 143.59,60.86 143.59,61.39 PC_NO2.11 | 133.1,114.73 v78.51,114.73 | v133.1,107.97 133.27,107.8 133.27,100.86 131.5,99.09 129.54,99.09 128.3,100.33 128.3,101.04 PC_AN9.5 | 133.1,114.73 v133.1,114.55
  Bottom 0.152: v78.51,114.73 v78.51,71.53 | v133.1,114.55 v133.1,107.97
M_SETPCN5  (via drill 0.35)
  Top 0.152: v85.45,68.5 84.91,68.5 83.84,67.44 83.84,66.9 PC_AN2.4 | v116.56,67.08 120.83,67.08 v122.43,68.68 | v125.09,71.35 125.09,71.7 125.63,72.24 125.63,72.77 PC_AN8.12 | v145.9,59.61 145.9,61.39 PC_NO2.9
  Route2 0.152: v85.45,68.5 85.98,68.5 87.4,67.08 v116.56,67.08 | 124.92,71.17 v122.43,68.68 | v145.9,59.61 145.9,58.37 143.76,56.24 141.99,56.24 130.43,67.79 128.3,67.79 124.92,71.17 | 124.92,71.17 v125.09,71.35
M_SETPCN6  (via drill 0.35)
  Top 0.152: PC_AN2.10 85.09,74.02 v85.62,74.55 | v128.83,68.5 128.83,67.44 128.3,66.9 PC_AN8.5 | v143.59,57.12 144.65,56.06 144.65,55.35 PC_NO2.7
  Route2 0.152: v85.62,74.55 93.62,74.55 94.69,75.62 129.18,75.62 134.87,81.31 135.59,81.31 135.94,80.95 135.94,80.24 133.1,77.39 133.1,72.77 130.43,70.1 | v128.83,68.5 130.43,70.1 | v143.59,57.12 130.61,70.1 130.43,70.1
M_SETPCN7  (via drill 0.35)
  Top 0.152: v83.84,75.26 83.84,72.95 PC_AN2.11 | v118.16,89.48 118.69,89.48 121.36,86.82 124.38,86.82 125.63,85.57 125.63,84.51 PC_AN7.12 | v139.14,53.75 141.28,53.75 142.16,54.63 142.16,55.35 PC_NO2.5
  Route2 0.152: v84.2,92.86 106.78,92.86 110.16,89.48 v118.16,89.48 | v139.14,53.75 131.32,53.75 120.29,64.77 v117.98,64.77
  Bottom 0.152: v83.84,75.26 84.2,75.62 v84.2,92.86 | v117.98,64.77 117.63,65.13 117.63,72.95 118.87,74.19 118.87,88.77 v118.16,89.48
M_SETPCN8  (via drill 0.35)
  Top 0.152: v132.21,58.55 132.92,57.84 139.14,57.84 139.68,57.3 139.68,55.35 PC_NO2.3 | v131.85,75.79 131.85,76.15 131.5,76.5 131.5,79.35 130.07,80.77 129.18,80.77 128.3,79.88 128.3,78.28 PC_AN7.5 | v98.78,64.59 97.36,63.17 96.65,63.17 95.4,64.41 95.4,66.73 PC_AN3.3
  Route15 0.152: v101.62,68.5 102.34,67.79 116.56,67.79 124.38,75.62 131.67,75.62 v131.85,75.79
  Bottom 0.152: v132.21,58.55 132.21,75.44 v131.85,75.79 | v98.78,64.59 101.62,67.44 v101.62,68.5
M_SETPCN9  (via drill 0.35)
  Top 0.152: v97,63.88 96.65,64.24 96.65,66.73 PC_AN3.4 | v135.41,70.81 137.36,70.81 138.07,71.53 138.96,71.53 139.68,72.24 139.68,72.77 PC_NO1.14 | v127.05,91.26 125.81,92.51 125.81,95.71 PC_AN6.12
  Route2 0.152: v127.05,91.26 129.01,89.31 129.9,89.31 135.94,83.26 137.01,83.26 140.03,80.24 140.03,79.53 144.12,75.44 144.65,75.44 145.01,75.08 145.01,74.37 141.81,71.17 135.76,71.17 v135.41,70.81
  Route15 0.152: v97,63.88 100.02,63.88 101.27,62.64 104.83,62.64 105.72,61.75 106.25,61.75 109.8,58.19 112.29,58.19 113.72,56.77 121.89,56.77 135.41,70.28 v135.41,70.81
M_SETPCN10  (via drill 0.35)
  Top 0.152: v122.25,80.59 122.25,78.99 118.52,75.26 99.49,75.26 97.89,73.66 97.89,72.95 PC_AN3.10 | v126.69,86.11 128.12,87.53 128.12,89.48 PC_AN6.5 | v142.88,74.73 143.41,74.19 143.41,72.95 PC_NO1.11
  Route2 0.152: v122.25,80.59 122.25,81.66 v126.69,86.11 131.5,86.11 v142.88,74.73
M_SETPCN11  (via drill 0.35)
  Top 0.152: v122.43,76.68 121.36,76.68 119.58,74.91 106.78,74.91 102.34,70.46 98.42,70.46 96.65,72.24 96.65,72.77 PC_AN3.11 | v132.21,77.04 135.41,77.04 137.01,75.44 138.07,75.44 | 138.07,75.44 144.65,75.44 145.9,74.19 145.9,72.95 PC_NO1.9 | v138.07,103.71 139.68,105.31 139.68,107.09 PC_AN5.12 | 138.07,75.44 v138.07,75.08
  Route15 0.152: v122.43,76.68 125.98,76.68 126.34,77.04 v132.21,77.04
  Bottom 0.152: v138.07,75.08 v138.07,103.71
M_SETPCN12
  Top 0.152: PC_AN4.11 111.76,62.1 113.36,63.7 126.69,63.7 126.87,63.88 138.25,63.88 138.43,64.06 142.7,64.06 144.65,66.02 144.65,66.73 PC_NO1.7 144.83,66.9 144.83,67.44 149.1,71.7 149.1,90.73 148.57,91.26 148.57,99.26 144.83,103 144.83,107.09 PC_AN5.8
M_USBDM
  Top 0.152: FT232.16 17.7,16.76 17.17,16.76 13.26,12.85 13.26,8.76 X2.2
M_USBDP
  Top 0.152: X2.3 13.97,10.19 17.7,13.92 17.7,16.05 FT232.15
N$1  (via drill 0.35)
  Top 0.152: v12.01,37.74 11.48,37.21 11.48,36.14 SE_JK1.15 | v19.66,40.59 22.33,40.59 23.22,39.7 26.59,39.7 26.77,39.52 30.15,39.52 32.99,36.68 32.99,36.14 SE_AN3.9 | v19.3,57.3 17.88,57.3 16.64,56.06 16.64,55.35 SE_JK2.6
  Route2 0.152: v12.01,37.74 14.15,37.74 16.28,39.88 18.95,39.88 v19.66,40.59
  Bottom 0.152: v19.3,57.3 19.3,40.95 v19.66,40.59
N$2  (via drill 0.35)
  Top 0.152: v16.46,24.59 10.24,24.59 FT232.1 | v18.06,38.46 16.64,37.03 16.64,36.14 SE_JK1.11 | v26.24,19.61 26.77,19.61 27.84,18.54 27.84,18.01 SE_N01.3 | v30.51,53.21 30.51,55.35 SE_JK3.5
  Route15 0.152: v30.51,53.21 30.51,52.5 18.06,40.06 v18.06,38.46
  Bottom 0.152: v16.46,24.59 17.88,26.01 18.59,26.01 | 18.59,26.01 18.59,37.92 v18.06,38.46 | v26.24,19.61 19.84,26.01 18.59,26.01
N$3  (via drill 0.35)
  Top 0.152: v17.88,26.72 18.41,26.72 21.97,23.16 21.97,19.43 24.99,16.41 25.88,16.41 26.59,17.12 26.59,17.83 SE_N01.2 | v17.88,34.01 17.88,35.97 SE_JK1.10 | SE_JK3.6 31.75,53.75 v32.11,53.39
  Route15 0.152: v32.11,53.39 32.11,51.44 17.88,37.21 v17.88,34.01
  Bottom 0.152: v17.88,34.01 v17.88,26.72
N$4
  Top 0.152: SE_JK12.13 13.97,73.48 13.08,74.37 9.7,74.37 7.21,71.88 7.21,36.14 10.06,33.3 10.06,30.1 SE_JK1.1
N$5  (via drill 0.35)
  Top 0.152: v24.28,35.61 27.84,32.05 27.84,30.1 SE_AN3.2 | v24.46,54.1 24.46,54.46 25.35,55.35 SE_JK3.1 | v32.99,59.79 32.99,61.39 SE_JK3.10
  Route2 0.152: v32.99,59.79 30.15,59.79 v24.46,54.1
  Bottom 0.152: v24.28,35.61 24.46,35.79 v24.46,54.1
N$6
  Top 0.152: SE_JK3.11 31.75,59.61 30.51,58.37 29.08,58.37 26.77,56.06 26.77,55.35 SE_JK3.2
N$7
  Top 0.152: M_OR1.3 41.17,30.1 41.17,31.7 40.28,32.59 34.24,32.59 34.06,32.41 30.33,32.41 30.15,32.59 29.44,32.59 28.02,34.01 28.02,35.97 SE_AN3.13
N$8
  Top 0.152: SE_JK4.15 26.77,72.77 26.77,70.81 27.66,69.93 33.35,69.93 34.95,71.53 34.95,74.19 33.53,75.62 33.17,75.62 31.75,77.04 SE_JK9.6 31.75,78.82 29.26,81.31 18.95,81.31 16.64,78.99 16.64,78.28 SE_JK5.6
N$9
  Top 0.152: 28.73,74.55 30.33,76.15 30.33,78.1 SE_JK9.5 | 28.73,74.55 28.02,73.84 28.02,72.95 SE_JK4.14 | 28.73,74.55 27.66,75.62 22.5,75.62 22.15,75.97 19.3,75.97 19.13,75.79 17.7,75.79 17.35,76.15 16.64,76.15 15.39,77.39 15.39,78.1 SE_JK5.5
N$11  (via drill 0.35)
  Top 0.152: v11.3,79.88 11.3,78.28 SE_JK5.2 | v16.28,82.73 16.28,84.15 16.46,84.33 SE_JK5.11 16.64,84.51 16.64,85.04 18.41,86.82 29.97,86.82 31.75,85.04 SE_JK9.11
  Route2 0.152: v11.3,79.88 14.15,82.73 v16.28,82.73
N$12
  Top 0.152: SE_JK5.1 10.24,78.28 10.24,79.88 11.66,81.31 15.93,81.31 17.7,83.08 17.7,84.33 SE_JK5.10
N$13
  Top 0.152: 16.46,90.37 14.86,91.97 10.59,91.97 9.35,90.73 9.35,88.59 11.3,86.64 11.3,84.51 SE_JK5.15 | 16.46,90.37 16.46,89.66 SE_JK6.6 16.46,90.37 | SE_JK10.6 31.75,91.26 31.04,91.97 18.06,91.97 16.46,90.37
N$14  (via drill 0.35)
  Top 0.152: v40.11,82.19 40.11,81.31 39.39,80.59 39.39,78.28 SE_JK8.1 | v39.93,86.11 39.93,90.91 40.11,91.08 41.17,91.08 41.88,90.37 41.88,89.66 SE_AN1.2
  Bottom 0.152: v40.11,82.19 39.93,82.37 v39.93,86.11
N$15
  Top 0.152: 33.88,64.24 32.82,65.3 32.64,65.3 31.75,66.19 SE_JK4.6 | 33.88,64.24 34.95,63.17 34.95,53.92 33.53,52.5 23.57,52.5 23.04,53.04 23.04,55.35 26.59,58.9 26.59,61.39 SE_JK3.15 | 33.88,64.24 35.66,66.02 35.66,71.88 39.22,75.44 43.66,75.44 45.62,77.39 45.62,78.1 SE_JK8.6
N$16  (via drill 0.35)
  Top 0.152: 15.21,87.53 14.68,87 13.97,87 12.72,85.75 12.72,84.51 SE_JK5.14 | 15.21,87.53 15.21,89.48 SE_JK6.5 | v29.97,87.88 30.33,88.24 30.33,89.48 SE_JK10.5 | 15.21,87.53 v17.88,87.53
  Route2 0.152: v29.97,87.88 24.1,87.88 23.75,87.53 v17.88,87.53
N$17  (via drill 0.35)
  Top 0.152: v14.5,91.26 11.12,91.26 10.24,90.37 10.24,89.66 SE_JK6.1 | v17.35,94.11 17.35,95.35 SE_JK6.10 | v32.11,93.57 32.99,94.46 32.99,95.71 SE_JK10.10
  Route2 0.152: v14.5,91.26 v17.35,94.11 18.41,93.04 30.51,93.04 31.04,93.57 v32.11,93.57
N$18  (via drill 0.35)
  Top 0.152: SE_JK6.14 12.72,95.88 12.72,96.77 14.86,98.91 14.86,100.69 SE_JK7.5 15.39,101.22 15.39,101.93 16.28,102.82 v18.77,102.82 | v30.15,99.44 30.33,99.62 30.33,101.04 SE_JK11.5
  Route2 0.152: v30.15,99.44 26.77,102.82 v18.77,102.82
N$19
  Top 0.152: 20.19,109.93 20.19,106.38 19.66,105.84 18.59,105.84 17.88,106.55 17.88,107.09 SE_JK7.10 | 20.19,109.93 20.19,110.11 19.48,110.82 11.84,110.82 9.35,108.33 9.35,106.02 10.06,105.31 10.06,101.22 SE_JK7.1 | 20.19,109.93 31.57,109.93 32.99,108.51 32.99,107.26 SE_JK11.10
N$20  (via drill 0.35)
  Top 0.152: v11.66,97.84 11.48,97.66 11.48,95.88 SE_JK6.15 | v16.28,99.44 16.28,100.86 16.46,101.04 SE_JK7.6 | SE_JK11.6 31.75,99.62 v31.57,99.44
  Route2 0.152: v11.66,97.84 13.26,99.44 v16.28,99.44 17.35,98.37 30.15,98.37 31.22,99.44 v31.57,99.44
N$21  (via drill 0.35)
  Top 0.152: 16.28,106.38 16.46,106.55 16.46,107.09 SE_JK7.11 16.28,106.38 | 16.28,106.38 15.75,105.84 15.57,105.84 11.48,101.75 11.48,101.22 SE_JK7.2 | SE_JK11.11 31.75,108.69 v31.57,108.86 | v24.46,105.13 17.53,105.13 16.28,106.38
  Route2 0.152: v31.57,108.86 28.91,106.2 25.53,106.2 v24.46,105.13
N$22
  Top 0.152: SE_AN1.1 SE_JK8.15
N$23  (via drill 0.35)
  Top 0.152: v27.3,79.88 26.42,79.88 25.53,78.99 25.53,78.28 SE_JK9.1 | v46.51,93.93 46.51,95.35 46.86,95.71 SE_AN1.9
  Route2 0.152: v27.3,79.88 29.44,79.88 43.48,93.93 v46.51,93.93
N$24
  Top 0.152: SE_JK3.14 28.02,61.57 28.02,62.99 30.33,65.3 30.33,66.73 SE_JK4.5 30.51,66.9 30.51,67.44 32.46,69.39 33.35,69.39 35.31,71.35 35.31,72.59 38.51,75.79 42.6,75.79 44.37,77.57 44.37,78.1 SE_JK8.5
N$25  (via drill 0.35)
  Top 0.152: v25.53,68.5 25.53,66.9 SE_JK4.1 | v29.79,74.55 30.51,74.55 31.22,75.26 31.93,75.26 32.99,74.19 32.99,72.95 SE_JK4.10 | v46.86,82.73 46.86,84.33 SE_JK8.10
  Route2 0.152: v25.53,68.5 25.53,69.39 26.77,70.64 26.77,71.53 v29.79,74.55 38.68,83.44 46.15,83.44 v46.86,82.73
N$26  (via drill 0.35)
  Top 0.152: v26.77,68.5 26.77,66.9 SE_JK4.2 | v31.57,74.55 31.57,73.13 31.75,72.95 SE_JK4.11 | v45.8,82.73 45.8,84.33 SE_JK8.11
  Route2 0.152: v26.77,68.5 26.77,69.39 31.57,74.19 v31.57,74.55 37.62,74.55 v45.8,82.73
N$27  (via drill 0.35)
  Top 0.152: v26.77,82.02 26.77,84.33 SE_JK9.15 | v44.2,99.44 44.91,99.44 47.22,97.13 47.57,97.13 48.11,96.6 48.11,95.88 SE_AN1.8
  Route15 0.152: v44.2,99.44 v26.77,82.02
N$28
  Top 0.152: SE_AN1.3 43.31,89.48 43.31,88.95 44.02,88.24 46.15,88.24 46.86,88.95 46.86,89.48 SE_AN1.6
N$29  (via drill 0.35)
  Top 0.152: v11.12,87.88 11.3,88.06 11.3,89.48 SE_JK6.2 | v10.77,93.22 15.04,93.22 15.21,93.04 30.51,93.04 31.75,94.28 SE_JK10.11 | v16.28,94.11 16.46,94.28 16.46,95.71 SE_JK6.11
  Route15 0.152: v16.28,94.11 15.75,94.11 14.86,93.22 v10.77,93.22
  Bottom 0.152: v11.12,87.88 10.77,88.24 v10.77,93.22
N$30
  Top 0.152: SE_AN1.5 45.8,89.66 45.8,95.71 SE_AN1.10
N$31
  Top 0.152: SE_JK10.15 26.77,95.88 26.77,96.6 28.55,98.37 41.17,98.37 43.13,96.42 43.13,95.88 SE_AN1.12
N$32  (via drill 0.35)
  Top 0.152: v23.57,34.9 26.59,31.88 26.59,30.1 SE_AN3.1 | v14.5,108.86 12.37,108.86 11.48,107.97 11.48,107.26 SE_JK7.15
  Bottom 0.152: v23.57,34.9 18.95,39.52 18.95,56.59 18.59,56.95 18.59,101.4 16.99,103 16.99,109.22 16.64,109.58 14.5,109.58 v14.5,108.86
N$33  (via drill 0.35)
  Top 0.152: 24.64,94.64 24.64,97.49 26.42,99.26 26.77,99.26 27.84,100.33 27.84,101.04 SE_JK11.3 27.84,101.22 27.84,103.35 26.95,104.24 26.42,104.24 24.64,106.02 24.64,108.86 25.35,109.58 28.73,109.58 29.08,109.22 29.08,107.26 SE_JK11.13 | 24.64,94.64 25.88,93.4 28.55,93.4 29.08,93.93 29.08,95.71 SE_JK10.13 | 42.06,80.06 42.06,82.55 43.13,83.62 43.13,84.33 SE_JK8.13 | 42.06,80.06 42.06,78.28 SE_JK8.3 | 29.62,30.99 29.97,31.34 31.04,31.34 31.75,30.63 SE_AN3.5 | 29.62,30.99 29.26,30.63 29.26,30.1 SE_AN3.3 | v23.39,80.59 27.66,80.59 28.02,80.24 28.02,78.28 SE_JK9.3 | v23.39,88.24 24.1,87.53 26.59,87.53 27.84,88.77 27.84,89.48 SE_JK10.3 | v29.62,82.73 29.26,83.08 29.26,84.33 SE_JK9.13 | 29.62,30.99 24.99,35.61 24.99,35.97 23.57,37.39 v22.15,37.39 | v40.11,80.06 42.06,80.06 | 24.64,94.64 24.28,94.64 v23.39,93.75
  Route2 0.152: v29.62,82.73 25.53,82.73 v23.39,80.59
  Route15 0.152: v40.11,80.06 32.28,80.06 v29.62,82.73
  Bottom 0.152: v22.15,37.39 21.08,38.46 21.08,40.95 22.33,42.19 22.33,79.53 v23.39,80.59 v23.39,88.24 v23.39,93.75
N$34  (via drill 0.35)
  Top 0.152: v42.6,99.44 42.06,99.97 42.06,101.04 SE_AN2.2 | v42.6,91.26 43.48,91.26 44.37,90.37 44.37,89.66 SE_AN1.4
  Bottom 0.152: v42.6,99.44 42.6,93.75 42.42,93.57 42.42,91.44 v42.6,91.26
N$35
  Top 0.152: SE_AN2.1 40.64,99.97 41.88,98.73 42.6,98.73 44.37,96.95 44.37,95.88 SE_AN1.11
N$36
  Top 0.152: SE_JK12.15 11.48,72.77 11.48,70.81 12.72,69.57 12.72,66.9 SE_JK12.3
N$37
  Top 0.152: SE_JK12.12 15.21,72.77 15.21,72.24 13.97,70.99 SE_JK12.4 13.97,66.19 16.46,63.7 20.9,63.7 21.62,62.99 21.62,60.5 19.48,58.37 10.24,58.37 7.57,55.7 7.57,36.32 12.55,31.34 13.26,31.34 13.97,30.63 SE_JK1.4 13.97,29.39 15.21,28.14 17.53,28.14 24.1,21.57 27.66,21.57 29.26,19.96 29.26,18.01 SE_N01.4
N$38  (via drill 0.35)
  Top 0.152: M_OR1.2 39.93,29.92 39.93,29.21 37.97,27.25 24.99,27.25 23.57,28.68 22.86,28.68 18.59,32.94 15.21,32.94 12.72,35.43 12.72,35.97 SE_JK1.14 12.72,36.14 12.72,38.1 12.37,38.46 11.12,38.46 8.28,41.3 v8.28,50.55 | v14.68,56.95 15.21,56.41 15.21,55.35 SE_JK2.5
  Route2 0.152: v8.28,50.55 v14.68,56.95
N$39
  Top 0.152: SE_AN3.8 34.24,36.14 34.24,36.86 30.86,40.23 27.13,40.23 22.33,45.03 22.33,50.72 20.55,52.5 12.37,52.5 10.24,54.63 10.24,55.35 SE_JK2.1
N$40
  Top 0.152: PC_JK1.2 93.98,104.06 96.47,106.55 96.47,107.09 PC_JK1.13
N$41  (via drill 0.35)
  Top 0.152: SE_JK2.3 12.55,55.35 12.55,56.06 11.48,57.12 9.53,57.12 8.99,56.59 8.99,41.12 10.77,39.34 13.26,39.34 13.97,38.63 SE_JK1.13 13.97,35.43 16.1,33.3 18.24,33.3 19.13,34.19 v22.15,34.19 | v30.33,34.37 30.33,35.97 SE_AN3.11
  Route2 0.152: v30.33,34.37 24.1,34.37 23.93,34.19 v22.15,34.19
N$42  (via drill 0.35)
  Top 0.152: v35.31,30.1 38.68,30.1 M_OR1.1 | v10.41,40.77 10.41,41.3 9.35,42.37 9.35,56.41 9.7,56.77 10.59,56.77 11.3,56.06 11.3,55.35 SE_JK2.2
  Route2 0.152: v35.31,30.1 22.86,30.1 16.1,36.86 11.3,36.86 10.41,37.74 v10.41,40.77
N$43  (via drill 0.35)
  Top 0.152: SE_AN2.5 45.72,99.69 45.85,99.57 v46.32,99.57 | v26.69,108.84 26.69,107.23 SE_JK11.15
  Route2 0.152: v46.32,99.57 45,99.57 40.09,104.47 24.19,104.47 23.8,104.86 23.8,106.67 25.97,108.84 v26.69,108.84
N$44  (via drill 0.35)
  Top 0.152: v25.53,103.53 25.53,101.22 SE_JK11.1 | v25.53,111 43.84,111 46.86,107.97 46.86,107.26 SE_AN2.9
  Bottom 0.152: v25.53,111 v25.53,103.53
N$45  (via drill 0.35)
  Top 0.152: v42.06,103.53 43.13,102.46 43.13,101.22 SE_AN2.3 | v42.06,105.31 42.06,107.09 SE_AN2.13 | PC_AN5.2 138.43,101.75 141.45,104.78 142.16,104.78 v142.88,105.49
  Route15 0.152: v142.88,105.49 139.85,105.49 126.16,119.18 55.93,119.18 v42.06,105.31
  Bottom 0.152: v42.06,105.31 v42.06,103.53
N$46
  Top 0.152: SE_AN2.12 43.31,107.09 43.31,106.38 43.84,105.84 44.91,105.84 45.62,106.55 45.62,107.09 SE_AN2.10
N$47  (via drill 0.35)
  Top 0.152: v20.9,60.86 20.55,60.86 20.02,61.39 19.13,61.39 SE_JK2.9 | v21.26,110.64 24.64,110.64 24.99,110.29 31.93,110.29 32.64,109.58 42.77,109.58 44.37,107.97 44.37,107.26 SE_AN2.11
  Bottom 0.152: v20.9,60.86 21.26,61.21 v21.26,110.64
N$48  (via drill 0.35)
  Top 0.152: v49.71,101.04 49.71,100.51 47.93,98.73 46.15,98.73 44.55,100.33 44.55,101.04 SE_AN2.4 | v135.41,101.22 137.01,101.22 PC_AN5.1
  Route15 0.152: v49.71,101.04 50.24,101.04 50.95,101.75 51.66,101.75 60.55,110.64 83.67,110.64 85.8,112.78 113.72,112.78 125.27,101.22 v135.41,101.22
N$49  (via drill 0.35)
  Top 0.152: v20.55,61.92 19.48,62.99 16.1,62.99 15.39,62.28 15.39,61.57 SE_JK2.12 | v136.12,100.51 136.12,100.15 136.65,99.62 138.96,99.62 139.68,100.33 139.68,101.04 PC_AN5.3
  Route15 0.152: v20.55,61.92 23.93,65.3 23.93,77.93 28.91,82.91 28.91,83.08 47.93,102.11 50.95,102.11 67.31,118.47 118.87,118.47 134.34,103 134.34,102.29 134.7,101.93 135.76,101.93 136.12,101.57 v136.12,100.51
N$50
  Top 0.152: PC_JK2.3 95.22,89.48 95.22,88.95 94.51,88.24 91.67,88.24 87.05,92.86 85.27,92.86 84.56,93.57 84.56,100.15 82.6,102.11 79.4,102.11 78.87,102.64 78.87,103.71 82.96,107.8 91.31,107.8 92.2,108.69 94.34,108.69 95.22,107.8 95.22,107.26 PC_JK1.14
N$51
  Top 0.152: PC_JK2.2 93.98,91.26 96.47,93.75 96.47,95.71 PC_JK2.13
N$52
  Top 0.152: PC_JK3.3 95.4,78.28 95.4,78.99 98.42,82.02 101.98,82.02 103.58,83.62 103.58,90.91 101.98,92.51 101.98,94.28 102.34,94.64 102.34,96.95 100.74,98.55 96.11,98.55 95.4,97.84 95.4,95.88 PC_JK2.14
N$53
  Top 0.152: PC_JK3.2 93.98,80.24 96.47,82.73 96.47,84.33 PC_JK3.13
N$54  (via drill 0.35)
  Top 0.152: v108.74,68.86 109.09,68.5 109.09,66.9 PC_JK4.3 | v95.4,82.73 95.4,84.33 PC_JK3.14
  Route15 0.152: v108.74,68.86 95.4,82.19 v95.4,82.73
N$55
  Top 0.152: PC_JK4.2 108.03,66.9 108.03,69.75 110.34,72.06 110.34,72.77 PC_JK4.13
N$56  (via drill 0.35)
  Top 0.152: v107.31,71.35 108.2,71.35 109.09,72.24 109.09,72.77 PC_JK4.14 | v107.31,99.26 108.03,99.26 109.09,100.33 109.09,101.04 PC_JK5.3
  Bottom 0.152: v107.31,99.26 v107.31,71.35
N$57
  Top 0.152: PC_JK5.2 108.03,101.22 108.03,104.06 110.34,106.38 110.34,107.09 PC_JK5.13
N$58
  Top 0.152: PC_JK6.3 109.27,89.66 109.27,90.37 111.94,93.04 118.52,93.04 118.87,93.4 118.87,95.35 115.67,98.55 106.96,98.55 104.83,100.69 104.83,102.11 109.09,106.38 109.09,107.09 PC_JK5.14
N$59
  Top 0.152: PC_JK6.2 108.03,89.66 108.03,91.62 110.34,93.93 110.34,95.71 PC_JK6.13
N$60  (via drill 0.35)
  Top 0.152: v108.03,81.31 109.09,80.24 109.09,78.28 PC_JK7.3 | v108.03,92.69 108.03,93.93 109.09,95 109.09,95.71 PC_JK6.14
  Bottom 0.152: v108.03,92.69 v108.03,81.31
N$61  (via drill 0.35)
  Top 0.152: v71.93,34.19 72.29,33.83 72.29,32.59 BR_NO2.5 | v64.29,65.48 64.29,71.53 63.75,72.06 | 63.75,72.06 61.44,74.37 59.31,74.37 58.42,73.48 BR_OR2.10 | v139.14,82.73 139.68,83.26 139.68,84.33 PC_AN11.12 | v64.29,72.41 63.93,72.06 63.75,72.06
  Route2 0.152: v97,87.88 94.51,87.88 86.51,79.88 73.71,79.88 66.24,72.41 v64.29,72.41
  Route15 0.152: v71.93,34.19 63.58,42.55 v63.58,43.08 | v139.14,82.73 137.54,82.73 136.65,83.62 135.41,83.62 129.36,89.66 129.36,94.46 129.01,94.82 98.07,94.82 94.87,91.62 94.87,90.02 v97,87.88
  Bottom 0.152: v63.58,43.08 64.29,43.79 v64.29,65.48
N$62  (via drill 0.35)
  Top 0.152: v104.29,99.62 101.09,99.62 100.38,100.33 100.38,101.04 PC_JK1.7 | v135.05,102.64 138.61,102.64 142.16,106.2 142.16,107.09 PC_AN5.10
  Route2 0.152: v104.29,99.62 106.6,99.62 109.09,102.11 134.52,102.11 v135.05,102.64
N$63  (via drill 0.35)
  Top 0.152: v97.18,102.82 96.65,102.29 96.65,101.22 PC_JK1.4 | v137.19,98.91 139.5,98.91 140.92,100.33 140.92,101.04 PC_AN5.4
  Route2 0.152: v97.18,102.82 98.42,102.82 102.34,98.91 103.94,98.91 104.29,98.55 119.23,98.55 121.89,101.22 134.34,101.22 136.65,98.91 v137.19,98.91
N$64  (via drill 0.35)
  Top 0.152: v110.69,109.4 105.18,109.4 103.05,107.26 101.62,107.26 PC_JK1.9 | v134.87,104.06 136.65,104.06 137.72,103 138.43,103 140.92,105.49 140.92,107.09 PC_AN5.11
  Route2 0.152: v110.69,109.4 128.47,109.4 133.81,104.06 v134.87,104.06
N$65  (via drill 0.35)
  Top 0.152: v117.09,91.62 121.36,87.35 125.45,87.35 125.81,87.71 125.81,89.48 PC_AN6.3 | v114.96,112.6 111.05,108.69 105,108.69 101.8,105.49 98.96,105.49 97.89,106.55 97.89,107.09 PC_JK1.12
  Bottom 0.152: v117.09,91.62 114.96,93.75 v114.96,112.6
N$66  (via drill 0.35)
  Top 0.152: v102.51,87.71 101.62,87.71 100.38,88.95 100.38,89.48 PC_JK2.7 | v126.69,87.17 126.69,89.31 126.87,89.48 PC_AN6.4
  Route2 0.152: v102.51,87.71 105.72,87.71 106.25,87.17 v126.69,87.17
N$67  (via drill 0.35)
  Top 0.152: v95.58,91.26 96.47,90.37 96.47,89.66 PC_JK2.4 | v128.65,94.11 128.65,95.35 128.3,95.71 PC_AN6.10
  Route15 0.152: v95.58,91.26 96.29,91.26 99.49,94.46 128.3,94.46 v128.65,94.11
N$68
  Top 0.152: PC_JK2.9 101.62,95.71 101.62,91.62 103.23,90.02 103.23,87.17 102.87,86.82 95.22,86.82 94.87,87.17 92.91,87.17 90.6,84.86 90.6,77.57 92.56,75.62 118.34,75.62 119.23,76.5 119.23,79.7 120.83,81.31 132.92,81.31 133.81,82.19 133.81,88.59 129.01,93.4 128.3,93.4 127.05,94.64 127.05,95.71 PC_AN6.11
N$69  (via drill 0.35)
  Top 0.152: v97.36,91.26 97.71,91.62 97.71,95.71 PC_JK2.12 | v123.67,80.59 124.74,80.59 125.63,79.7 125.63,78.28 PC_AN7.3
  Route15 0.152: v97.36,91.26 97.71,91.26 105.72,83.26 121.01,83.26 v123.67,80.59
N$70  (via drill 0.35)
  Top 0.152: v104.65,76.33 101.62,76.33 100.38,77.57 100.38,78.1 PC_JK3.7 | v126.69,76.33 126.69,77.93 126.87,78.1 PC_AN7.4
  Route2 0.152: v104.65,76.33 117.27,76.33 117.63,75.97 126.34,75.97 v126.69,76.33
N$71  (via drill 0.35)
  Top 0.152: v98.6,76.33 97.71,76.33 96.65,77.39 96.65,78.1 PC_JK3.4 | v128.65,82.73 128.65,83.97 PC_AN7.10
  Route2 0.152: v98.6,76.33 103.58,76.33 104.29,77.04 117.09,77.04 117.8,76.33 121.01,76.33 123.85,79.17 125.09,79.17 v128.65,82.73
N$72  (via drill 0.35)
  Top 0.152: v102.87,84.33 101.62,84.33 PC_JK3.9 | v118.16,82.02 123.85,82.02 124.03,81.84 125.09,81.84 126.87,83.62 126.87,84.33 PC_AN7.11
  Route2 0.152: v102.87,84.33 115.85,84.33 v118.16,82.02
N$73  (via drill 0.35)
  Top 0.152: v101.62,82.73 98.78,82.73 97.89,83.62 97.89,84.33 PC_JK3.12 | v116.2,69.04 118.52,69.04 118.87,69.39 124.74,69.39 125.63,68.5 125.63,66.9 PC_AN8.3
  Route15 0.152: v101.62,82.73 102.51,82.73 v116.2,69.04
N$74
  Top 0.152: PC_JK4.7 114.43,66.73 114.43,66.02 116.38,64.06 125.63,64.06 126.87,65.3 126.87,66.73 PC_AN8.4
N$75
  Top 0.152: PC_JK4.4 110.52,66.9 110.52,68.86 111.4,69.75 125.81,69.75 128.12,72.06 128.12,72.77 PC_AN8.10
N$76
  Top 0.152: PC_JK4.9 115.67,72.95 118.16,72.95 120.47,75.26 125.27,75.26 126.87,73.66 126.87,72.95 PC_AN8.11
N$77  (via drill 0.35)
  Top 0.152: PC_JK4.12 111.76,72.24 113.54,70.46 v121.54,70.46 | v121.54,99.8 122.61,99.8 122.78,99.62 124.92,99.62 125.63,100.33 125.63,101.04 PC_AN9.3
  Bottom 0.152: v121.54,99.8 v121.54,70.46
N$78
  Top 0.152: PC_JK5.7 114.43,101.04 114.43,100.33 115.85,98.91 124.56,98.91 124.74,99.09 125.81,99.09 126.87,100.15 126.87,101.04 PC_AN9.4
N$79
  Top 0.152: PC_JK5.4 110.52,101.22 110.52,101.75 112.47,103.71 123.67,103.71 123.85,103.53 125.98,103.53 128.12,105.66 128.12,107.09 PC_AN9.10
N$80
  Top 0.152: PC_JK5.9 115.67,107.09 120.83,107.09 124.03,103.89 125.81,103.89 127.05,105.13 127.05,107.09 PC_AN9.11
N$81  (via drill 0.35)
  Top 0.152: PC_JK5.12 111.76,108.33 117.09,113.66 132.39,113.66 133.81,112.24 133.81,100.15 v135.05,98.91 | v135.05,91.62 135.05,89.13 137.01,87.17 137.9,87.17 139.68,88.95 139.68,89.48 PC_AN10.3
  Bottom 0.152: v135.05,91.62 v135.05,98.91
N$82
  Top 0.152: PC_JK6.7 114.25,89.66 114.25,91.8 115.14,92.69 118.69,92.69 121.72,95.71 121.72,97.66 122.61,98.55 124.74,98.55 124.92,98.73 129.01,98.73 130.61,97.13 133.1,97.13 137.72,92.51 143.05,92.51 143.41,92.86 146.43,92.86 148.74,90.55 148.74,78.82 145.72,75.79 137.19,75.79 134.52,78.46 134.52,84.15 137.19,86.82 139.32,86.82 140.92,88.42 140.92,89.48 PC_AN10.4
N$83  (via drill 0.35)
